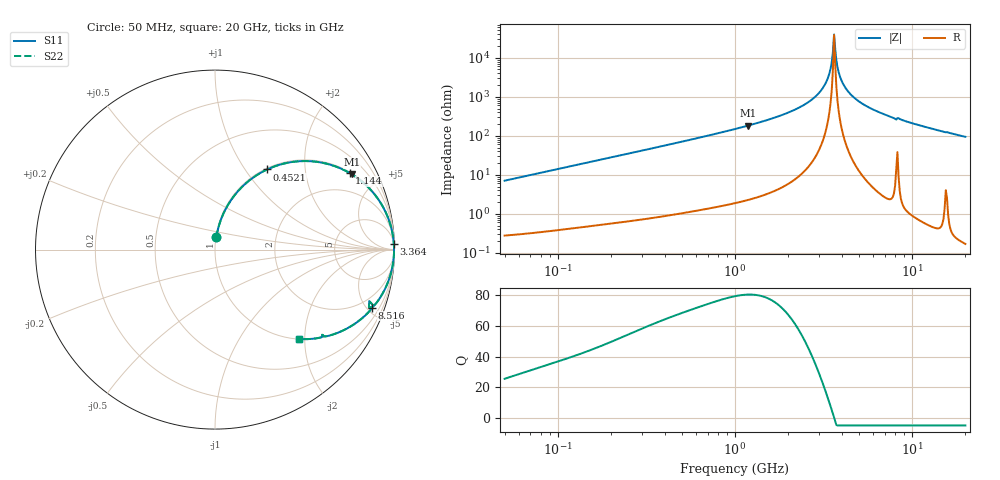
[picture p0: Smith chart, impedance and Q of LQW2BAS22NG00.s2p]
!Murata Part Number: LQW2BAS22NG00
!These Parameters are Measured in Series Mode Connection
!  o--[Z]--o
!Port1  Port2
!  o-------o
!Freq. Start=50[MHz] Stop=20[GHz], 401[Steps]
# Hz S RI R 50
!Freq.(Hz) S11(Real) S11(Imag) S21(Real) S21(Imag) S12(Real) S12(Imag) S22(Real) S22(Imag)
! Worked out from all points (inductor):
!   401 points, 50 MHz to 20 GHz, reference 50 ohm
!   read as one part in series: L = 22.4 nH near 51.52 MHz
!   highest Q = 80.5 at 1.179 GHz (marker M1), where L = 24.5 nH
!   self-resonance near 3.626 GHz
!   S11 on the Smith chart (normalised r, x): 50 MHz: 1.01, +0.14; 452.1 MHz: 1.02, +1.27; 1.144 GHz: 1.04, +3.49; 3.364 GHz: 6, +65; 8.516 GHz: 1.08, -5.39; 20 GHz: 1.00, -1.88
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5e7  0.00768 0.0698  0.9923 -0.0698  0.9923 -0.0698  0.00768 0.0698
1.364002e8  0.0392 0.1826  0.9608 -0.1826  0.9608 -0.1826  0.0392 0.1826
3.721004e8  0.2172 0.4045  0.7828 -0.4045  0.7828 -0.4045  0.2172 0.4045
4.520922e8  0.2904 0.4465  0.7096 -0.4465  0.7096 -0.4465  0.2904 0.4465
1e9  0.687 0.4575  0.313 -0.4575  0.313 -0.4575  0.687 0.4575
1.144317e9  0.7506 0.4265  0.2494 -0.4265  0.2494 -0.4265  0.7506 0.4265
1.179116e9  0.7639 0.4185  0.2361 -0.4185  0.2361 -0.4185  0.7639 0.4185
1.962148e9  0.9322 0.2441  0.0678 -0.2441  0.0678 -0.2441  0.9322 0.2441
2.728004e9  0.9838 0.1142  0.0162 -0.1142  0.0162 -0.1142  0.9838 0.1142
3.121702e9  0.9937 0.0604  0.00634 -0.0604  0.00634 -0.0604  0.9937 0.0604
3.364474e9  0.9965 0.0305  0.00348 -0.0305  0.00348 -0.0305  0.9965 0.0305
3.466789e9  0.9971 0.0186  0.00285 -0.0186  0.00285 -0.0186  0.9971 0.0186
3.519108e9  0.9974 0.0126  0.00265 -0.0126  0.00265 -0.0126  0.9974 0.0126
3.626126e9  0.9975 0.000615  0.00245 -0.000615  0.00245 -0.000615  0.9975 0.000615
3.736399e9  0.9975 -0.0114  0.00255 0.0114  0.00255 0.0114  0.9975 -0.0114
3.850025e9  0.9971 -0.0233  0.00293 0.0233  0.00293 0.0233  0.9971 -0.0233
3.967106e9  0.9964 -0.0353  0.00361 0.0353  0.00361 0.0353  0.9964 -0.0353
4.405649e9  0.9917 -0.0773  0.00829 0.0773  0.00829 0.0773  0.9917 -0.0773
5.433528e9  0.9711 -0.1613  0.0289 0.1613  0.0289 0.1613  0.9711 -0.1613
7.442007e9  0.907 -0.2868  0.093 0.2868  0.093 0.2868  0.907 -0.2868
8.516016e9  0.8753 -0.3233  0.1247 0.3233  0.1247 0.3233  0.8753 -0.3233
2e10  0.4691 -0.4981  0.5309 0.4981  0.5309 0.4981  0.4691 -0.4981
